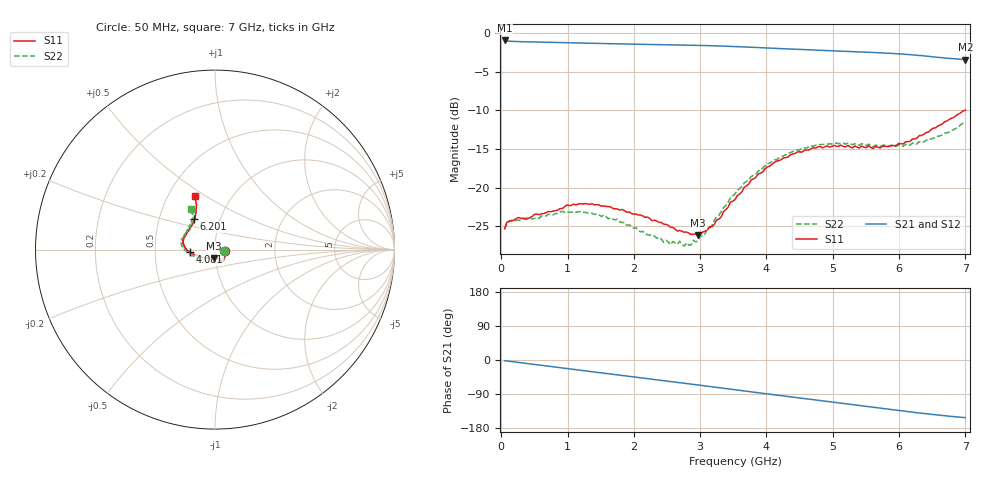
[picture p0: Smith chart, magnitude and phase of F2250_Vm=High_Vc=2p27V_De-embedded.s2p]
! Integrated Device Technology
! Corporate Headquarters
! 6024 Silver Creek Valley Road
! San Jose, CA 95138  USA
! Phone:  1-408-284-8200
! Toll Free:  1-800-223-1366
! Webpage:  http://www.idt.com/
! Timing and RF Division
! 515 Groton Road, Suite 102
! Westford, MA 01886-6024
! Device:  F2250
! Description: Voltage Variable RF Attenuator
! Frequency:  50.0 -  6000.00 MHz
! Package:  3x3 mm Thin QFN Plastic Package: 16 pin
! Ports:  2 RF, 3 DC
!  Pin  1  = GND
!  Pin  2  = NC
!  Pin  3  = RF1  = Port 1
!  Pin  4  = NC
!  Pin  5  = GND
!  Pin  6  = GND
!  Pin  7  = GND
!  Pin  8  = GND
!  Pin  9  = NC
!  Pin 10  = RF2  = Port 2
!  Pin 11  = NC
!  Pin 12  = GND
!  Pin 13  = GND
!  Pin 14  = VCNTRL
!  Pin 15  = VDD
!  Pin 16  = VMODE
! Vcntrl:  2.270 Volts
! Vmode:  +3.300 Volts
! Vdd:  +3.30  Volts
! Current:  1.316 mA
! Data:  The device was measured on a the F2250 evaluation board which has
!  individual transmission lines to the RF pins.  Data was collected
!  using a calibrated network analyzer.  The evaluation board was
!  de-embedded using a TRL calibration technique.
!  The reference plane is the edge of the package pin.
! Misc:  SN 10
!  Action Tracker AT0258
! Date Measured:  2014-11-26
! Date:  2015-10-15  MJV
! Note:
!  Integrated Device Technology supplies this data as a sample of measured
!  data at the package pin for this product.  Your particular data for this
!  product may vary.
!  Data was taken at 25 degrees C.
!  Integrated Device Technology reserves the right to change this data at anytime.
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# GHz S dB R 50
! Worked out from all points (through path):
!   201 points, 50 MHz to 7 GHz, reference 50 ohm
!   highest |S21| = -0.91 dB at 50 MHz (marker M1); lowest = -3.4 dB at 7 GHz (marker M2)
!   group delay of S21, straight-line fit = 61.1 ps
!   lowest |S11| = -26.2 dB at 2.969 GHz (marker M3), VSWR 1.10, Z = 49.3 - j4.82 ohm
!   |S11| at or under -10 dB: start of sweep to 6.986 GHz
!   |S22| runs from -27.6 to -11.5 dB; largest |S21 - S12| = 0.0019
!   S11 on the Smith chart (normalised r, x): 50 MHz: 1.11, -0.02; 4.081 GHz: 0.75, -0.02; 6.201 GHz: 0.75, +0.27; 7 GHz: 0.68, +0.45
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0.05  -25.30 -10.2  -0.91 -1.8  -0.91 -1.8  -25.45 -10.6
0.1195  -24.39 -9.9  -1.01 -3.2  -1.01 -3.2  -24.35 -8.7
0.91875  -22.75 -49.0  -1.20 -21.0  -1.19 -21.1  -23.08 -50.3
1.2315  -22.14 -56.8  -1.26 -27.9  -1.26 -27.9  -23.20 -60.8
1.75275  -22.79 -63.7  -1.35 -39.1  -1.35 -39.1  -24.11 -67.4
2.37825  -24.53 -63.5  -1.44 -52.8  -1.45 -52.8  -26.47 -67.4
2.552  -25.16 -68.3  -1.47 -56.7  -1.47 -56.7  -27.41 -73.9
2.691  -25.57 -76.0  -1.49 -59.8  -1.49 -59.8  -26.96 -81.4
2.7605  -25.81 -78.2  -1.51 -61.3  -1.51 -61.3  -27.61 -85.8
2.969  -26.20 -95.7  -1.55 -66.0  -1.55 -66.0  -26.89 -104.8
3.21225  -24.79 -125.7  -1.60 -71.5  -1.60 -71.5  -24.24 -129.8
3.4555  -21.91 -146.8  -1.68 -77.0  -1.68 -77.0  -21.35 -145.0
3.525  -21.57 -151.1  -1.70 -78.5  -1.70 -78.6  -20.82 -148.3
3.76825  -19.02 -163.6  -1.79 -84.0  -1.79 -84.0  -18.59 -159.3
4.081  -17.01 -174.8  -1.92 -91.0  -1.92 -91.0  -16.64 -171.1
4.4285  -15.59 176.7  -2.05 -98.6  -2.06 -98.6  -15.14 178.9
4.7065  -14.82 169.7  -2.15 -104.8  -2.15 -104.8  -14.63 173.2
5.054  -14.67 161.6  -2.28 -112.5  -2.28 -112.5  -14.23 166.1
5.85325  -14.65 135.6  -2.58 -130.0  -2.58 -130.1  -14.64 147.3
6.20075  -13.69 124.0  -2.79 -137.7  -2.79 -137.8  -14.23 138.3
6.54825  -12.25 116.0  -3.06 -144.7  -3.06 -144.8  -13.56 126.9
7  -9.96 111.0  -3.39 -152.1  -3.40 -152.2  -11.53 120.7
